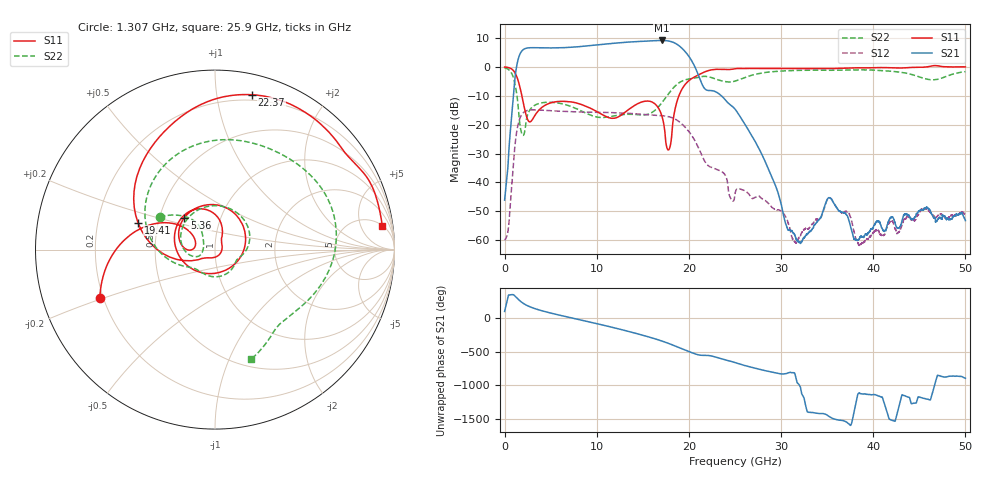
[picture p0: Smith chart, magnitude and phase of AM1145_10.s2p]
!Agilent Technologies,E8364B,MY43040894,A.07.50.67
!Agilent E8364B: A.07.50.67
!Date: Monday, November 15, 2021 11:31:44
!Correction: S11(Full 2 Port(1,2))
!S21(Full 2 Port(1,2))
!S12(Full 2 Port(1,2))
!S22(Full 2 Port(1,2))
!S2P File: Measurements: S11, S21, S12, S22:
# Hz S  dB  R 50
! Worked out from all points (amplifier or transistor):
!   6401 points, 10 MHz to 50 GHz, reference 50 ohm
!   highest |S21| = 9.2 dB at 17.05 GHz (marker M1)
!   |S21| within 3 dB of that: 2.112 GHz to 19.34 GHz (17.23 GHz wide, 161 % of centre)
!   unconditionally stable (mu >= 1): start of sweep to 45.75 GHz
!   at 8.336 GHz: K = 1.41, MAG = 7.5 dB, |S12| = -15.6 dB
!   at 25 GHz: K = 34.21, MAG = -3.7 dB, |S12| = -43.9 dB
!   at 50 GHz: K = -281.75, MSG = -1.0 dB, |S12| = -51.2 dB
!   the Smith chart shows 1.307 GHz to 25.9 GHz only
!   S11 on the Smith chart (normalised r, x): 1.307 GHz: 0.19, -0.19; 5.36 GHz: 0.67, +0.25; 19.41 GHz: 0.38, +0.15; 22.37 GHz: 0.15, +1.26; 25.9 GHz: 5, +12
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1e7  -0.00 -12.4  -46.18 102.2  -60.08 166.8  -0.25 -16.7
1.306616e9  -3.16 -157.3  0.12 -51.5  -22.78 162.4  -8.94 149.4
1.853381e9  -9.54 153.4  5.47 -119.2  -16.57 88.2  -22.94 152.4
2.704773e9  -19.01 165.5  6.68 175.1  -14.95 17.2  -15.12 178.3
3.938902e9  -14.31 170.3  6.67 117.3  -14.94 -43.4  -12.47 118.4
5.360492e9  -12.16 133.8  6.63 66.4  -15.22 -94.4  -12.30 69.1
8.34427e9  -13.00 57.2  7.13 -27.7  -15.61 176.5  -15.24 -1.4
1.075785e10  -16.76 -20.4  7.89 -104.3  -15.75 106.8  -17.49 -29.2
1.309332e10  -15.65 -138.4  8.57 176.3  -16.00 36.6  -16.43 -73.7
1.510854e10  -11.94 144.3  8.94 102.0  -16.46 -27.3  -16.62 -125.4
1.667854e10  -14.12 90.0  9.19 37.7  -16.77 -82.2  -13.90 -153.4
1.704565e10  -16.70 76.1  9.22 21.0  -16.86 -96.5  -12.50 -161.8
1.8436e10  -15.62 -158.0  8.38 -50.4  -17.93 -158.4  -6.82 148.6
1.941237e10  -6.85 160.7  5.99 -105.1  -20.26 153.3  -4.66 105.1
2.080272e10  -3.12 116.6  -1.00 -178.2  -26.45 86.9  -3.72 52.2
2.237271e10  -1.04 76.5  -8.16 158.3  -34.71 55.0  -3.58 -3.6
2.5005e10  -0.56 25.3  -14.58 56.6  -43.86 7.0  -4.89 -56.1
2.590326e10  -0.52 7.8  -18.91 19.1  -42.68 -44.7  -3.84 -71.7
3.333927e10  -0.55 -111.0  -56.44 30.3  -54.65 48.1  -1.08 160.3
4.167354e10  -0.23 157.1  -53.38 -46.5  -54.35 -53.2  -1.37 65.9
4.659443e10  0.49 125.5  -52.33 48.0  -51.88 -119.5  -4.43 -86.4
5e10  0.05 103.3  -53.27 -178.2  -51.23 -153.5  -1.61 151.1
